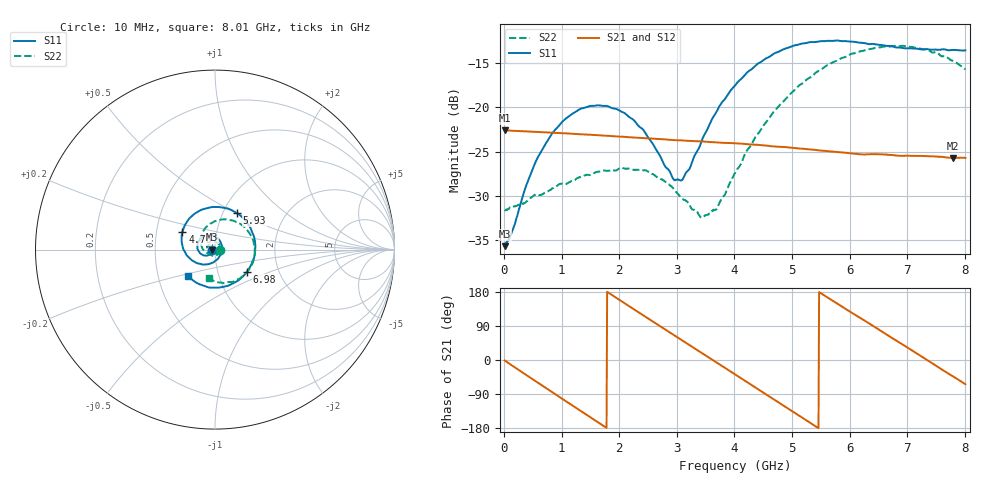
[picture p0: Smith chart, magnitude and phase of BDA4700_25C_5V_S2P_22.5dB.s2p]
!Agilent Technologies,E5071B,MY42404982,A.09.10
!Date: Mon Oct 20 13:37:43 2025
!Data & Calibration Information:
!Freq	S11:SOLT2(ON)	S21:SOLT2(ON)	S12:SOLT2(ON)	S22:SOLT2(ON)
# Hz S RI R 50
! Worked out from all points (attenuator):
!   801 points, 10 MHz to 8.01 GHz, reference 50 ohm
!   highest |S21| = -22.58 dB at 20 MHz (marker M1); lowest = -25.7 dB at 7.79 GHz (marker M2)
!   lowest |S11| = -35.7 dB at 10 MHz (marker M3), VSWR 1.03, Z = 48.4 - j0.111 ohm
!   |S11| at or under -10 dB: start of sweep to end of sweep
!   |S22| runs from -32.5 to -13.0 dB; largest |S21 - S12| = 0.00056
!   S11 on the Smith chart (normalised r, x): 10 MHz: 0.97, -0.00; 4.76 GHz: 0.68, +0.14; 5.93 GHz: 1.16, +0.50; 6.98 GHz: 1.38, -0.36; 8.01 GHz: 0.71, -0.22
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1e7  -0.0163 -0.00115  0.0743 -0.00161  0.0743 -0.00168  0.0262 -0.000854
2e7  -0.0167 -0.00187  0.0743 -0.00285  0.0743 -0.00301  0.0261 -0.00109
6.2e8  -0.0431 -0.0334  0.0328 -0.0647  0.0327 -0.0647  0.0115 -0.0297
1.01e9  -0.0795 -0.0235  -0.0152 -0.0698  -0.0153 -0.0698  -0.0155 -0.0336
1.35e9  -0.0984 0.00892  -0.0509 -0.0486  -0.051 -0.0486  -0.0365 -0.0176
2.08e9  -0.0474 0.0804  -0.0596 0.0329  -0.0597 0.033  -0.0294 0.0344
2.68e9  0.028 0.0473  -0.00243 0.0662  -0.00243 0.0662  0.0138 0.0372
2.94e9  0.0384 0.00832  0.0259 0.06  0.0259 0.0599  0.0258 0.0233
3.09e9  0.0351 -0.0163  0.0401 0.0512  0.0398 0.0513  0.0284 0.0114
3.41e9  0.0029 -0.0617  0.0601 0.0228  0.0601 0.0228  0.0203 -0.0127
3.54e9  -0.0178 -0.0743  0.0632 0.00897  0.0633 0.00885  0.0126 -0.0213
3.7e9  -0.0496 -0.0821  0.0628 -0.00829  0.0628 -0.00845  -0.00127 -0.027
4.01e9  -0.1142 -0.0682  0.0494 -0.0385  0.0495 -0.0384  -0.0333 -0.0263
4.76e9  -0.1811 0.0992  -0.022 -0.0558  -0.0218 -0.0559  -0.08 0.0614
5.35e9  -0.0644 0.2256  -0.0566 -0.0108  -0.0566 -0.011  -0.015 0.1496
5.93e9  0.1224 0.2036  -0.039 0.0392  -0.0391 0.0391  0.116 0.1545
6.37e9  0.2128 0.0841  -0.00345 0.0542  -0.00352 0.0541  0.1993 0.079
6.68e9  0.2217 -0.0265  0.0241 0.0482  0.0242 0.0482  0.221 -0.00237
6.98e9  0.1773 -0.1239  0.0435 0.0307  0.0436 0.0305  0.2054 -0.0828
7.37e9  0.0626 -0.204  0.0529 -0.00225  0.0529 -0.0023  0.1349 -0.1633
7.79e9  -0.0877 -0.1926  0.0379 -0.0351  0.0379 -0.0352  0.02 -0.1825
8.01e9  -0.1502 -0.1477  0.0227 -0.0465  0.0229 -0.0466  -0.0331 -0.1606
